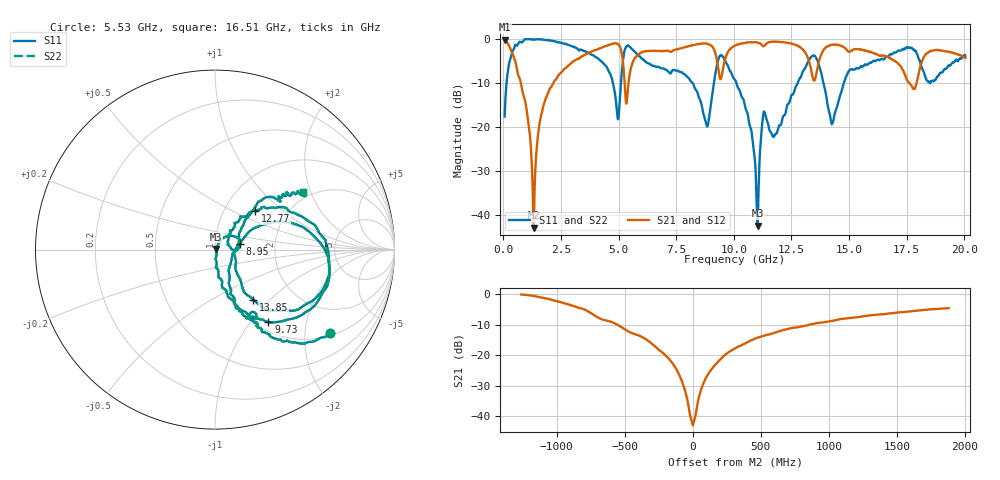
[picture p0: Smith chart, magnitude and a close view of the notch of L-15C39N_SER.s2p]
#	mhz	s	ma	r	50
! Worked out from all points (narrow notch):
!   1001 points, 50 MHz to 20.05 GHz, reference 50 ohm
!   highest |S21| = -0.16 dB at 50 MHz (marker M1); lowest = -43.0 dB at 1.31 GHz (marker M2)
!   notch at M2: 40.2 dB deep, 316 MHz wide at half that depth
!   lowest |S11| = -42.5 dB at 11.03 GHz (marker M3), VSWR 1.02, Z = 50.7 + j0.333 ohm
!   |S11| at or under -10 dB: 8.204 GHz to 9.136 GHz (931.5 MHz wide, 10.7 % of centre); 10.11 GHz to 12.78 GHz (2.668 GHz wide, 23.3 % of centre); 13.89 GHz to 14.77 GHz (888.3 MHz wide, 6.2 % of centre)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
!   |S22| runs from -42.5 to 0.0 dB; largest |S21 - S12| = 0
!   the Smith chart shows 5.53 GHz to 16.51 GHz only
!   S11 on the Smith chart (normalised r, x): 5.53 GHz: 1.07, -2.70; 8.95 GHz: 1.32, +0.08; 9.73 GHz: 1.14, -1.23; 12.77 GHz: 1.40, +0.67; 13.85 GHz: 1.26, -0.80; 16.51 GHz: 1.80, +1.76
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50  0.1308 79.3  0.9823 -6.8  0.9823 -6.8  0.1308 79.3
930  0.9876 5.2  0.2018 -81.2  0.2018 -81.2  0.9876 5.2
1310  0.9823 -5.3  0.0071 -7.1  0.0071 -7.1  0.9823 -5.3
1870  0.9722 -18.2  0.2187 71.4  0.2187 71.4  0.9722 -18.2
3390  0.7471 -44.0  0.629 41.8  0.629 41.8  0.7471 -44.0
4950  0.1287 -37.5  0.8781 -7.2  0.8781 -7.2  0.1287 -37.5
5530  0.7934 -36.0  0.4642 37.5  0.4642 37.5  0.7934 -36.0
6730  0.482 -60.6  0.7285 10.2  0.7285 10.2  0.482 -60.6
8950  0.1419 12.8  0.8606 -19.3  0.8606 -19.3  0.1419 12.8
9390  0.6399 -7.2  0.3601 -21.3  0.3601 -21.3  0.6399 -7.2
9730  0.5018 -53.6  0.6991 11.8  0.6991 11.8  0.5018 -53.6
10050  0.3437 -70.3  0.8398 2.4  0.8398 2.4  0.3437 -70.3
11030  0.00747 26.1  0.9137 -16.6  0.9137 -16.6  0.00747 26.1
11310  0.1497 21.2  0.8309 -16.1  0.8309 -16.1  0.1497 21.2
12770  0.3123 43.7  0.8339 -42.2  0.8339 -42.2  0.3123 43.7
13390  0.6343 -3.0  0.3994 -50.7  0.3994 -50.7  0.6343 -3.0
13850  0.3504 -52.7  0.7178 -9.8  0.7178 -9.8  0.3504 -52.7
14270  0.1095 -6.9  0.8599 -26.7  0.8599 -26.7  0.1095 -6.9
16510  0.5855 33.5  0.6469 -53.1  0.6469 -53.1  0.5855 33.5
16730  0.6412 31.6  0.6126 -57.0  0.6126 -57.0  0.6412 31.6
18030  0.5928 -20.5  0.4137 -6.4  0.4137 -6.4  0.5928 -20.5
20050  0.6428 7.9  0.609 -72.3  0.609 -72.3  0.6428 7.9
